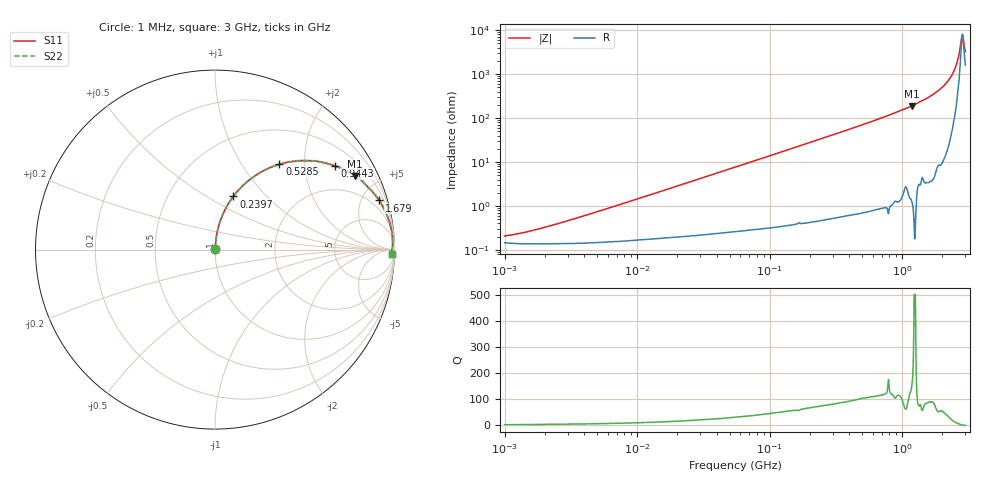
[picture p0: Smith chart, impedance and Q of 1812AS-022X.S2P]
!s-Parameter Generated by FASTRON Sdn. Bhd.
!FASTRON P/N : 1812AS-022X
!Keysight Technologies,E4991B,MY54100416,A.01.15
!Date created:  Fri Oct 13 13:55:39 2023
!Version  : Rev00  Fri Oct 13 13:55:39 2023
!Data & Calibration Information:
!Freq	S11	S21	S12	S22
!PortZ  Port1:50+j0  Port2:50+j0
!When reading, reference impedance value at option line is always used.
! Remarks : This data is being provided solely for informational purposes.
# Hz S dB R 50
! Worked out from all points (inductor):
!   1601 points, 1 MHz to 3 GHz, reference 50 ohm
!   read as one part in series: L = 23.3 nH near 2.846 MHz
!   highest Q = 150 at 1.183 GHz (marker M1), where L = 25.5 nH
!   self-resonance near 2.839 GHz
!   S11 on the Smith chart (normalised r, x): 1 MHz: 1.00, +0.00; 239.7 MHz: 1.01, +0.66; 528.5 MHz: 1.01, +1.49; 944.3 MHz: 1.03, +2.86; 1.679 GHz: 1.08, +6.65; 3 GHz: 33, -57
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1000000  -53.66 45.5  -0.01 -0.1  -0.01 -0.1  -53.66 45.5
1674325  -50.98 60.7  -0.01 -0.1  -0.01 -0.1  -50.98 60.7
3804036  -44.84 75.3  -0.01 -0.3  -0.01 -0.3  -44.84 75.3
1.447069e7  -33.74 83.8  -0.02 -1.2  -0.02 -1.2  -33.74 83.8
5.477226e7  -22.40 83.7  -0.05 -4.3  -0.05 -4.3  -22.40 83.7
1.109129e8  -16.41 80.1  -0.13 -8.7  -0.13 -8.7  -16.41 80.1
2.083556e8  -11.19 73.1  -0.38 -16.0  -0.38 -16.0  -11.19 73.1
2.396927e8  -10.08 70.9  -0.49 -18.3  -0.49 -18.3  -10.08 70.9
3.594878e8  -7.03 62.9  -1.01 -26.4  -1.01 -26.4  -7.03 62.9
5.284703e8  -4.51 52.9  -1.96 -36.5  -1.96 -36.5  -4.51 52.9
7.925923e8  -2.43 40.5  -3.74 -49.1  -3.74 -49.1  -2.43 40.5
9.443041e8  -1.77 34.8  -4.87 -54.7  -4.87 -54.7  -1.77 34.8
1.182785e9  -1.09 27.7  -6.64 -61.9  -6.64 -61.9  -1.09 27.7
1.67892e9  -0.40 16.7  -10.84 -72.7  -10.84 -72.7  -0.40 16.7
2.050964e9  -0.18 10.5  -14.76 -78.3  -14.76 -78.3  -0.18 10.5
2.371269e9  -0.09 6.0  -19.66 -81.1  -19.66 -81.1  -0.09 6.0
2.581816e9  -0.08 3.2  -24.93 -79.0  -24.93 -79.0  -0.08 3.2
2.647227e9  -0.08 2.4  -27.27 -76.0  -27.27 -76.0  -0.08 2.4
2.769173e9  -0.09 0.9  -34.21 -55.6  -34.21 -55.6  -0.09 0.9
2.825159e9  -0.10 0.3  -37.63 -24.1  -37.63 -24.1  -0.10 0.3
2.896736e9  -0.12 -0.5  -36.03 32.6  -36.03 32.6  -0.12 -0.5
3e9  -0.13 -1.5  -30.38 59.0  -30.38 59.0  -0.13 -1.5
